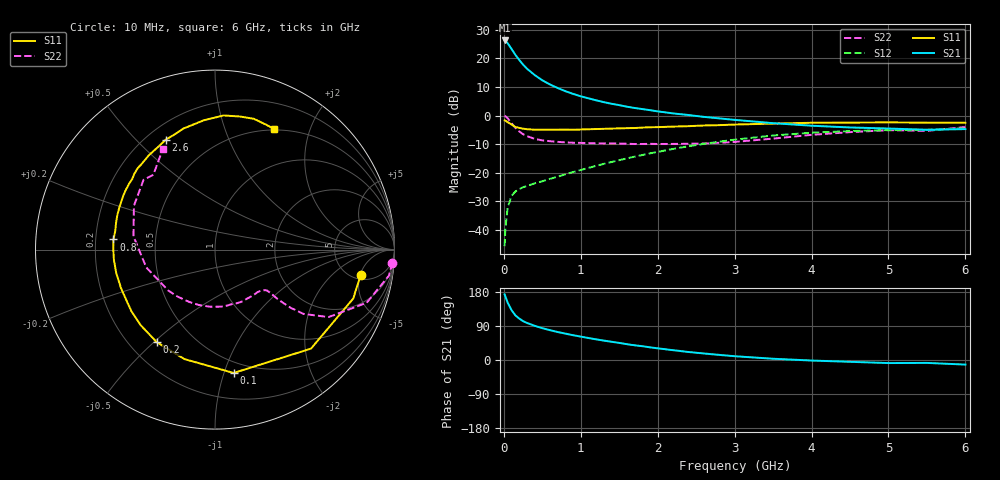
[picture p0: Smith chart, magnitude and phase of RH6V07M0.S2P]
! SIEMENS Small Signal Semiconductors
! BFR106
! Si NPN RF Bipolar Junction Transistor in SOT23
! VCE = 6 V  IC = 7 mA
! Common Emitter S-Parameters:  August  1996
# GHz  S  MA  R  50
!  f  S11  S21  S12  S22
! GHz  MAG  ANG  MAG  ANG  MAG  ANG  MAG  ANG
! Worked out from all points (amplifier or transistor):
!   36 points, 10 MHz to 6 GHz, reference 50 ohm
!   highest |S21| = 26.3 dB at 10 MHz (marker M1)
!   |S21| within 3 dB of that: start of sweep to 101.2 MHz
!   unconditionally stable (mu >= 1): 564.8 MHz to 1.886 GHz; 5.124 GHz to end of sweep
!   at 250 MHz: K = 0.59, MSG = 21.4 dB, |S12| = -25.1 dB
!   at 1.4 GHz: K = 1.11, MAG = 8.1 dB, |S12| = -16.2 dB
!   at 6 GHz: K = 1.01, MAG = -0.9 dB, |S12| = -4.5 dB
!   S11 on the Smith chart (normalised r, x): 10 MHz: 5.84, -5.11; 100 MHz: 0.41, -1.08; 200 MHz: 0.31, -0.51; 800 MHz: 0.28, +0.05; 2.6 GHz: 0.27, +0.61; 6 GHz: 0.49, +1.49
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0.01  0.8242 -9.8  20.61 173.1  0.0052 86.5  0.9902 -4.2
0.02  0.817 -19.5  20.37 167.8  0.0106 79.3  0.9801 -8.5
0.05  0.7683 -45.9  18.4 151.1  0.0247 67.4  0.8957 -19.3
0.1  0.6952 -81.4  14.68 131.7  0.0395 54.6  0.7363 -30.7
0.15  0.6333 -105.6  11.54 117.9  0.047 46.8  0.6098 -36.0
0.2  0.6091 -122.2  9.402 109.4  0.0518 44.3  0.5299 -37.6
0.25  0.5908 -134.4  7.781 102.5  0.0558 42.9  0.4723 -38.1
0.3  0.5783 -143.8  6.63 97.9  0.0589 43.9  0.4377 -38.3
0.4  0.5662 -157.4  5.128 90.3  0.0652 45.8  0.3919 -38.0
0.5  0.5655 -166.5  4.142 84.0  0.071 48.6  0.368 -38.2
0.6  0.5662 -174.1  3.5 78.7  0.0783 51.7  0.3566 -39.3
0.8  0.5688 174.3  2.673 69.6  0.094 56.4  0.3399 -43.0
1.1  0.5769 160.7  2.003 58.0  0.1215 61.1  0.3303 -51.1
1.3  0.5868 153.0  1.717 51.2  0.1431 62.4  0.3262 -57.5
1.6  0.6029 142.8  1.43 41.7  0.1786 63.1  0.3222 -68.8
2.2  0.6418 125.1  1.093 25.9  0.2612 59.4  0.3195 -95.4
2.6  0.6714 114.1  0.949 17.2  0.3198 54.4  0.3251 -116.4
3.5  0.7239 94.7  0.737 3.3  0.4487 39.2  0.3957 -165.5
4.5  0.7544 79.3  0.62 -4.8  0.5359 20.2  0.5135 151.6
5  0.7603 73.5  0.594 -8.1  0.5581 12.1  0.5564 135.7
5.5  0.7519 67.7  0.565 -7.7  0.5639 7.9  0.5403 129.5
6  0.7486 63.9  0.58 -12.1  0.599 -0.2  0.631 117.4
